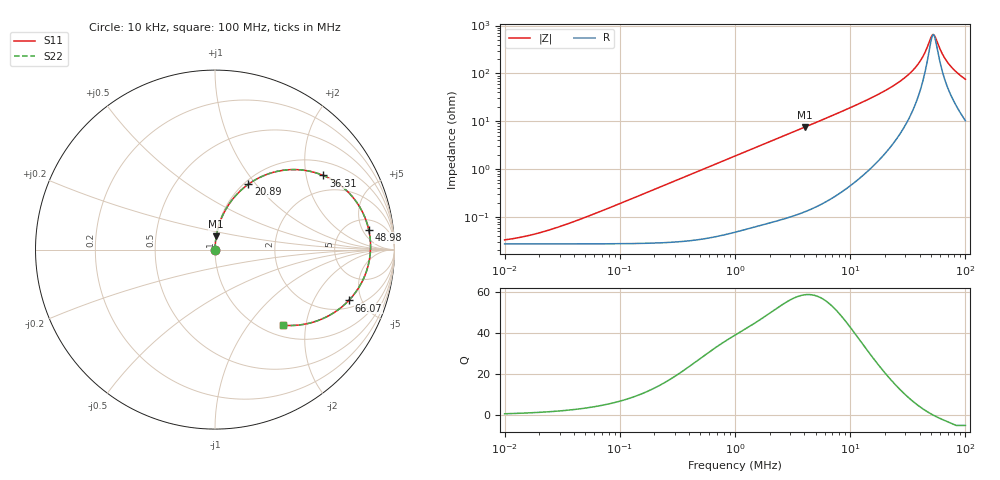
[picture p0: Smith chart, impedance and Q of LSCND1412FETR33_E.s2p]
! LSCND1412FETR33_E  S-PARAMETER MODEL  ( Standard Model )
! Model Generated by TAIYO YUDEN Corporation (http://www.ty-top.com)
! Version 1.0
! TAIYO YUDEN Control No. 231226
! Copyright(c) 2023 TAIYO YUDEN CO.,LTD. All Rights Reserved.
! Product Description (link to TY-COMPAS)
! https://ds.yuden.co.jp/TYCOMPAS/or/detail?pn=LSCND1412FETR33ME&u=M
! Products Name : Inductors
! Characteristics :
!  Inductance : 0.33 [uH] , SRF(min) : - [Hz] , DC Resistance(max) : 32 [mOhm]
!  Rated Current : Saturation  5.4 [A] (dL = 30 [%]), Temp Rise  3.7 [A] (dT = 40 [degC])
!  Case Size : 1.4 x 1.2 / 0.055 x 0.047 [mm/inch] , Thickness : 0.65 / 0.026 [mm/inch]
!  (Conditions: Temperature = 25 [degC] , DC Bias Current = 0 [A])
! External Node Assignments :
!  1  o---GGG---o  2
! GND o---------o GND
! Frequency Range : 10kHz  -  100MHz  [ 402 STEP ]
# MHz S RI R 50
! Freq[MHz].  S11 Real  S11 Imag  S21 Real  S21 Imag  S12 Real  S12 Imag  S22 Real  S22 Imag
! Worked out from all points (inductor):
!   401 points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, 10 kHz to 100 MHz, reference 50 ohm
!   read as one part in series: L = 299 nH near 43.65 kHz
!   highest Q = 58.7 at 4.074 MHz (marker M1), where L = 296 nH
!   self-resonance near 52.74 MHz
!   S11 on the Smith chart (normalised r, x): 10 kHz: 1.00, +0.00; 20.89 MHz: 1.05, +0.92; 36.31 MHz: 1.42, +2.52; 48.98 MHz: 8, +7; 66.07 MHz: 2.51, -3.90; 100 MHz: 1.20, -1.49
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0.01  0.000273 0.000188  0.9997 -0.000188  0.9997 -0.000188  0.000273 0.000188
0.019953  0.000273 0.000375  0.9997 -0.000375  0.9997 -0.000375  0.000273 0.000375
0.046774  0.000274 0.000879  0.9997 -0.000879  0.9997 -0.000879  0.000274 0.000879
0.218776  0.000304 0.00411  0.9997 -0.00411  0.9997 -0.00411  0.000304 0.00411
1  0.000828 0.0187  0.9992 -0.0187  0.9992 -0.0187  0.000828 0.0187
4.073803  0.00697 0.0751  0.993 -0.0751  0.993 -0.0751  0.00697 0.0751
4.677351  0.00898 0.0862  0.991 -0.0862  0.991 -0.0862  0.00898 0.0862
12.02264  0.0574 0.2194  0.9426 -0.2194  0.9426 -0.2194  0.0574 0.2194
16.2181  0.1076 0.2919  0.8924 -0.2919  0.8924 -0.2919  0.1076 0.2919
20.89296  0.1863 0.3644  0.8137 -0.3644  0.8137 -0.3644  0.1863 0.3644
21.87762  0.2062 0.3779  0.7938 -0.3779  0.7938 -0.3779  0.2062 0.3779
29.51209  0.3983 0.444  0.6017 -0.444  0.6017 -0.444  0.3983 0.444
36.30781  0.6035 0.413  0.3965 -0.413  0.3965 -0.413  0.6035 0.413
42.65795  0.7693 0.2901  0.2307 -0.2901  0.2307 -0.2901  0.7693 0.2901
45.70882  0.823 0.2068  0.177 -0.2068  0.177 -0.2068  0.823 0.2068
48.97788  0.8569 0.1099  0.1431 -0.1099  0.1431 -0.1099  0.8569 0.1099
51.28614  0.8662 0.0414  0.1338 -0.0414  0.1338 -0.0414  0.8662 0.0414
53.70318  0.8645 -0.0273  0.1355 0.0273  0.1355 0.0273  0.8645 -0.0273
58.88437  0.8304 -0.1561  0.1696 0.1561  0.1696 0.1561  0.8304 -0.1561
66.06934  0.7453 -0.2835  0.2547 0.2835  0.2547 0.2835  0.7453 -0.2835
79.43282  0.5729 -0.3957  0.4271 0.3957  0.4271 0.3957  0.5729 -0.3957
100  0.3779 -0.4212  0.6221 0.4212  0.6221 0.4212  0.3779 -0.4212
